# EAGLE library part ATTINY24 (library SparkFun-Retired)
Atmel 20-pin 2kB flash uC Retired
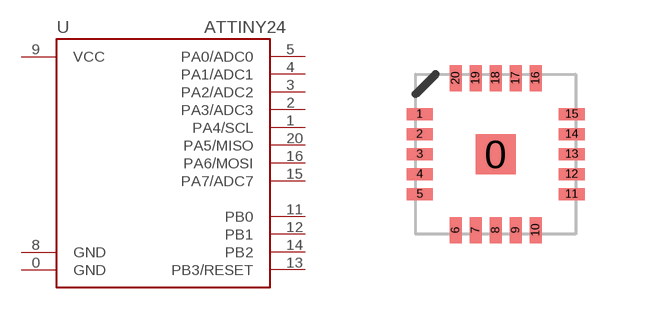
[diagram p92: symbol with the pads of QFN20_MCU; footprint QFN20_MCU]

Designator prefix -

## ATTINY24QFN  [QFN20_MCU]
0  GND
1  PA4/SCL
2  PA3/ADC3
3  PA2/ADC2
4  PA1/ADC1
5  PA0/ADC0
8  GND
9  VCC
11  PB0
12  PB1
13  PB3/RESET
14  PB2
15  PA7/ADC7
16  PA6/MOSI
20  PA5/MISO

## Footprint QFN20_MCU (pad centres in mm)
smd 1 x 1: 0 0,0
smd 0.65 x 0.3: 1 -1.9,1; 2 -1.9,0.5; 3 -1.9,0; 4 -1.9,-0.5; 5 -1.9,-1; 11 1.9,-1; 12 1.9,-0.5; 13 1.9,0; 14 1.9,0.5; 15 1.9,1
smd 0.3 x 0.65: 6 -1,-1.9; 7 -0.5,-1.9; 8 0,-1.9; 9 0.5,-1.9; 10 1,-1.9; 16 1,1.9; 17 0.5,1.9; 18 0,1.9; 19 -0.5,1.9; 20 -1,1.9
